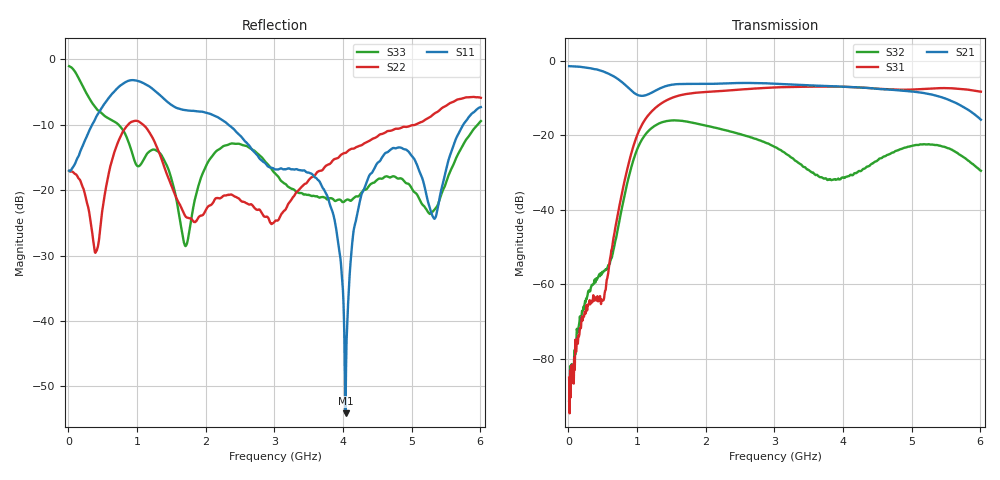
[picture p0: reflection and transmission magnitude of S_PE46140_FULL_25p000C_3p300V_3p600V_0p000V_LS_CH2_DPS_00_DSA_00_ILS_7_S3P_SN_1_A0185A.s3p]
! Device ID: PE46140_FULL
! File Path: z:\PE46140\MajorStates\25p000C\3p300\LS_CH2_DPS_00_DSA_00_ILS_7\PE46140_FULL_25p000C_3p300V_3p600V_0p000V_LS_CH2_DPS_00_DSA_00_ILS_7_S3P_SN_1_A0185A.s3p
! Serial: 1
! Lot: A0185A
! Temp: 25.000C
! VDD: 3.300
! VSS: 0.000
! Control_Hi: 3.600
! Control_Lo: 0.000
! Logic State: LS_CH2_DPS_00_DSA_00_ILS_7
! Port 1: RFIN
! Port 2: RFOUT1
! Port 3: RFOUT2
! ThroughPath:1-3
! IDD: 0.000314732
! ISS: -1.694e-007
! Comment:
#  Hz  S  RI  R  50
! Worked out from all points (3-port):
!   801 points, 10 MHz to 6.01 GHz, reference 50 ohm
!   strongest paths, dB at 10 MHz, 1.51 GHz, 3.01 GHz, 4.51 GHz, 6.01 GHz:
!     S21: -1.5, -6.5, -6.2, -7.6, -15.9
!     S31: -85.0, -10.0, -7.2, -7.5, -8.3
!     S32: -91.1, -16.0, -23.2, -26.6, -29.5
!   lowest |S11| = -54.1 dB at 4.037 GHz (marker M1), VSWR 1.00, Z = 49.8 + j0.0275 ohm
!   |S11| at or under -10 dB: start of sweep to 346.1 MHz; 2.329 GHz to 5.753 GHz (3.424 GHz wide, 84.7 % of centre)
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1e7  0.1401 -0.0109  0.842 -0.0246  3.22e-07 4.36e-07
     0.8418 -0.0244  0.14 -0.00675  -3.47e-05 4.03e-05
     5.09e-05 2.34e-05  -2.48e-05 -1.25e-05  0.8809 -0.0831
3.55e8  -0.016 -0.3218  0.4591 -0.6283  -0.000596 -0.000368
        0.4593 -0.6263  -0.00912 -0.0426  -0.000115 0.000986
        -0.000534 -0.000301  -0.000146 0.000974  -0.4042 -0.2107
1.165e9  -0.5852 0.224  -0.2047 -0.288  -0.1835 -0.0274
         -0.2049 -0.2885  0.2134 -0.1871  -0.00287 0.1136
         -0.1837 -0.0277  -0.003 0.1136  0.166 0.1008
1.705e9  -0.2851 0.2923  -0.4873 0.00283  0.2595 0.2415
         -0.4873 0.00299  0.0344 -0.0529  -0.0256 -0.1508
         0.2597 0.2418  -0.0254 -0.1511  -0.0365 -0.00755
3.01e9  0.0181 0.1427  0.409 0.2716  -0.378 -0.2183
        0.4088 0.2725  -0.0578 -0.00129  0.0619 -0.031
        -0.3783 -0.2184  0.062 -0.0312  0.125 -0.0491
3.7675e9  0.0253 0.0877  0.2753 -0.3638  -0.2302 0.3849
          0.2757 -0.3637  0.0774 0.1346  -0.0139 0.0214
          -0.2302 0.3846  -0.0139 0.0212  0.0823 -0.0209
4.0375e9  -0.00195 0.000277  0.0426 -0.4429  -0.00267 0.4456
          0.0432 -0.4432  0.1393 0.1326  0.0231 0.0149
          -0.00151 0.4452  0.0232 0.0147  0.0804 -0.022
4.3825e9  -0.1037 -0.0765  -0.2528 -0.3448  0.2624 0.3389
          -0.2529 -0.3453  0.2157 0.0992  0.0144 -0.0361
          0.2629 0.3383  0.0142 -0.036  0.1031 -0.0324
5.335e9  -0.0407 -0.0445  -0.1077 0.3256  0.3078 -0.2931
         -0.109 0.3256  0.3832 -0.0374  0.0124 0.073
         0.3079 -0.2926  0.0123 0.073  0.0701 0.0114
6.01e9  -0.2978 -0.3111  0.153 0.0484  -0.1974 -0.3264
        0.1537 0.0486  0.2471 -0.443  0.0276 -0.0183
        -0.199 -0.3275  0.0278 -0.0185  0.3119 0.1274
